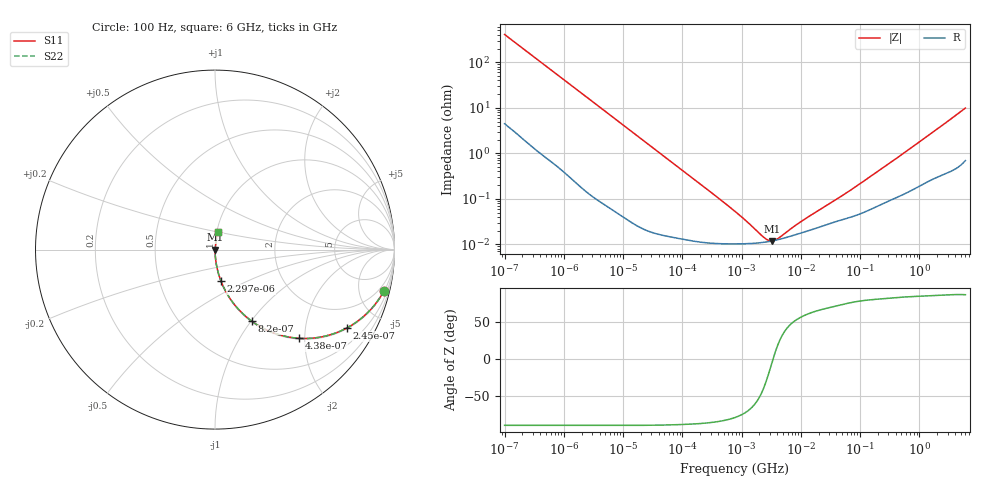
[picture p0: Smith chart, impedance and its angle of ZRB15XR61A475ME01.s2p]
!Murata Part Number: ZRB15XR61A475ME01
!These Parameters are Measured in Series Mode Connection
!Data Generated on Jun 10, 2025
!  o--ll--o
!Port1  Port2
!  o------o
!Operation Temp=25[degC], DC Bias Voltage=0[V]
!Freq. Start=100[Hz] Stop=6[GHz] 401[Steps]
# Hz S RI R 50
!Freq.(Hz) S11(Real) S11(Imag) S21(Real) S21(Imag) S12(Real) S12(Imag) S22(Real) S22(Imag)
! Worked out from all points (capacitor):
!   401 points, 100 Hz to 6 GHz, reference 50 ohm
!   read as one part in series: C = 3.88 uF near 109 Hz
!   lowest |Z| = 11.9 mohm at 3.246 MHz (marker M1)
!   series resonance near 3.408 MHz, so ESL is about 560 pH
!   S11 on the Smith chart (normalised r, x): 100 Hz: 1.09, -8.18; 245 Hz: 1.03, -3.36; 438 Hz: 1.02, -1.88; 820 Hz: 1.01, -1.01; 2.297 kHz: 1.00, -0.36; 6 GHz: 1.01, +0.20
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100  0.9414 -0.2296  0.0586 0.2296  0.0586 0.2296  0.9414 -0.2296
164  0.8602 -0.3416  0.1398 0.3416  0.1398 0.3416  0.8602 -0.3416
245  0.7364 -0.4356  0.2636 0.4356  0.2636 0.4356  0.7364 -0.4356
335  0.6013 -0.4848  0.3987 0.4848  0.3987 0.4848  0.6013 -0.4848
438  0.4705 -0.4943  0.5295 0.4943  0.5295 0.4943  0.4705 -0.4943
820  0.2057 -0.3995  0.7943 0.3995  0.7943 0.3995  0.2057 -0.3995
1227  0.105 -0.3021  0.895 0.3021  0.895 0.3021  0.105 -0.3021
2008  0.0428 -0.1982  0.9572 0.1982  0.9572 0.1982  0.0428 -0.1982
2297  0.0332 -0.1752  0.9668 0.1752  0.9668 0.1752  0.0332 -0.1752
7036  0.00407 -0.0593  0.9959 0.0593  0.9959 0.0593  0.00407 -0.0593
40335  0.000274 -0.0104  0.9997 0.0104  0.9997 0.0104  0.000274 -0.0104
774597  0.000102 -0.00052  0.9999 0.00052  0.9999 0.00052  0.000102 -0.00052
2372521  0.000111 -8.96e-05  0.9999 8.96e-05  0.9999 8.96e-05  0.000111 -8.96e-05
2837864  0.000115 -4.4e-05  0.9999 4.4e-05  0.9999 4.4e-05  0.000115 -4.4e-05
3245845  0.000118 -1.15e-05  0.9999 1.15e-05  0.9999 1.15e-05  0.000118 -1.15e-05
4246196  0.000128 5.09e-05  0.9999 -5.09e-05  0.9999 -5.09e-05  0.000128 5.09e-05
8311524  0.000164 0.00021  0.9998 -0.00021  0.9998 -0.00021  0.000164 0.00021
1.555665e7  0.000212 0.000403  0.9998 -0.000403  0.9998 -0.000403  0.000212 0.000403
5.960426e7  0.000373 0.00131  0.9996 -0.00131  0.9996 -0.00131  0.000373 0.00131
3.124326e8  0.000942 0.00594  0.9991 -0.00594  0.9991 -0.00594  0.000942 0.00594
1.873145e9  0.00386 0.0317  0.9961 -0.0317  0.9961 -0.0317  0.00386 0.0317
6e9  0.0163 0.0963  0.9837 -0.0963  0.9837 -0.0963  0.0163 0.0963
